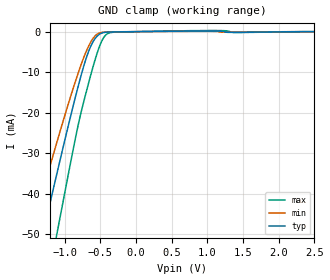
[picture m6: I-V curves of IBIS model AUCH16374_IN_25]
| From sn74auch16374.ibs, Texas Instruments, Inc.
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[Model]   AUCH16374_IN_25
Model_type  Input
Vinl=0.7
Vinh=1.7
| variable   typ   min   max
C_comp   2.66pF   2.05pF   3.11pF
[Temperature Range]   40   100   -40
| Ambient temperature   25   85   -40
[Voltage range]   2.5   2.3   2.7
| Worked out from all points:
|   GND clamp passes 1 mA (typ) near -0.54 V on its own axis
[GND Clamp]
| AUCH16374_IN_25
|   Voltage   I(typ)   I(min)   I(max)
-3.6V     -229mA     -190.7mA   -277mA
-1.48V    -63.46mA   -50.44mA   -84.23mA
-1.43V    -59.6mA    -47.27mA   -79.63mA
-1.295V   -49.23mA   -38.79mA   -67.19mA
-1.105V   -34.82mA   -27.12mA   -49.66mA
-830mV    -14.89mA   -11.31mA   -24.77mA
-720mV    -7.851mA   -5.889mA   -16.5mA
-620mV    -3.131mA   -2.167mA   -9.875mA
-520mV    -760.2uA   -408.2uA   -4.107mA
-430mV    -174.9uA   -99.91uA   -971.3uA
-310mV    -72.55uA   -46.67uA   -140.4uA
2.5V      355.7pA    563.3nA    -12.78nA
